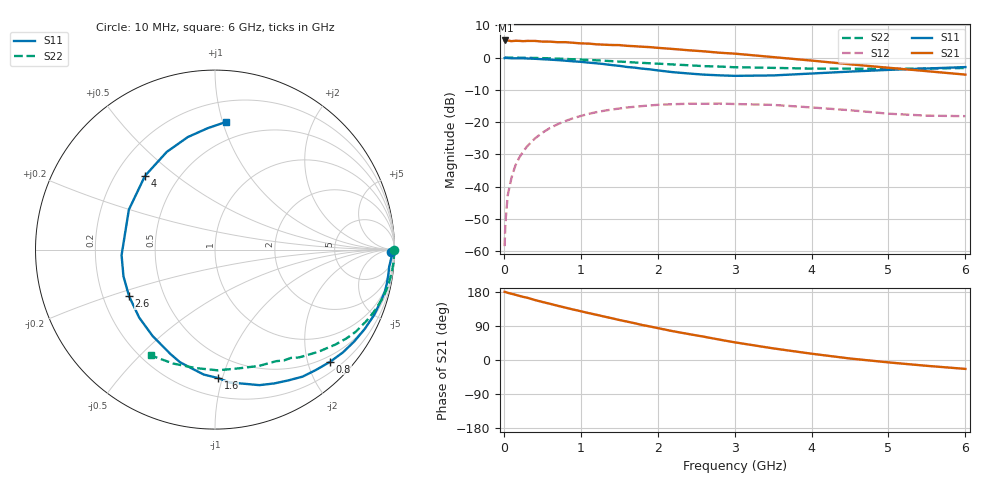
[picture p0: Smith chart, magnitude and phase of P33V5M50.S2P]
! SIEMENS Small Signal Semiconductors
! BFP181
! Si NPN RF Bipolar Junction Transistor in SOT143
! VCE = 3.5 V  IC = 0.5 mA
! Common Emitter S-Parameters:  March  1996
# GHz  S  MA  R  50
!  f  S11  S21  S12  S22
! GHz  MAG  ANG  MAG  ANG  MAG  ANG  MAG  ANG
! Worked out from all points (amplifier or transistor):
!   36 points, 10 MHz to 6 GHz, reference 50 ohm
!   highest |S21| = 5.3 dB at 20 MHz (marker M1)
!   |S21| within 3 dB of that: start of sweep to 2.383 GHz
!   unconditionally stable (mu >= 1): 3.779 GHz to end of sweep
!   at 250 MHz: K = 0.07, MSG = 17.1 dB, |S12| = -29.2 dB
!   at 1.4 GHz: K = 0.42, MSG = 10.0 dB, |S12| = -16.1 dB
!   at 6 GHz: K = 1.45, MAG = 2.4 dB, |S12| = -18.1 dB
!   S11 on the Smith chart (normalised r, x): 10 MHz: 72, -43; 800 MHz: 0.38, -2.41; 1.6 GHz: 0.33, -0.97; 2.6 GHz: 0.31, -0.23; 4 GHz: 0.32, +0.39; 6 GHz: 0.35, +1.02
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0.01  0.9798 -0.7  1.816 179.8  0.0012 93.0  0.9999 -0.2
0.02  0.9903 -1.2  1.842 179.5  0.0027 86.1  0.9995 -0.5
0.05  0.984 -2.5  1.839 177.4  0.0073 89.6  0.9983 -1.4
0.1  0.9752 -5.6  1.796 174.8  0.0139 85.5  0.9976 -2.7
0.15  0.9759 -8.3  1.821 172.2  0.0213 83.6  0.9971 -4.0
0.2  0.976 -11.1  1.816 169.3  0.0282 82.0  0.9951 -5.4
0.3  0.9687 -16.8  1.813 164.6  0.0419 78.4  0.9911 -8.1
0.4  0.9584 -22.3  1.812 158.5  0.0553 74.1  0.9869 -10.7
0.6  0.9292 -33.5  1.765 148.3  0.0813 66.2  0.9728 -15.9
0.8  0.8959 -44.2  1.733 138.2  0.104 58.8  0.9531 -20.8
1.1  0.8356 -60.7  1.648 123.9  0.1342 48.2  0.919 -27.8
1.5  0.7449 -83.7  1.562 105.6  0.1624 35.2  0.8669 -36.3
1.6  0.7158 -88.7  1.521 101.4  0.1687 32.5  0.8556 -38.1
1.9  0.6569 -107.3  1.452 88.5  0.1815 23.9  0.8159 -43.7
2.2  0.5939 -125.8  1.359 75.9  0.1895 16.4  0.7817 -48.7
2.6  0.5446 -151.6  1.25 61.5  0.1923 7.7  0.7368 -55.0
3  0.5214 -176.6  1.151 46.7  0.1909 -0.8  0.7087 -61.3
3.5  0.529 155.1  1.018 30.7  0.185 -8.9  0.693 -69.2
4  0.5665 133.5  0.899 16.6  0.169 -15.1  0.675 -78.5
4.5  0.607 116.3  0.787 3.9  0.153 -19.7  0.6728 -88.7
5.5  0.6775 93.5  0.616 -15.4  0.1261 -15.9  0.6763 -110.1
6  0.7133 85.2  0.545 -23.5  0.1238 -11.8  0.6894 -121.3
